FUNCTION "ASSE Y" : VOID
TITLE =GESTIONE SEGNALI DI STATO E COMANDO DELL'ASSE Y
VERSION : 0.1

BEGIN
NETWORK
TITLE =INS./DISIN.1
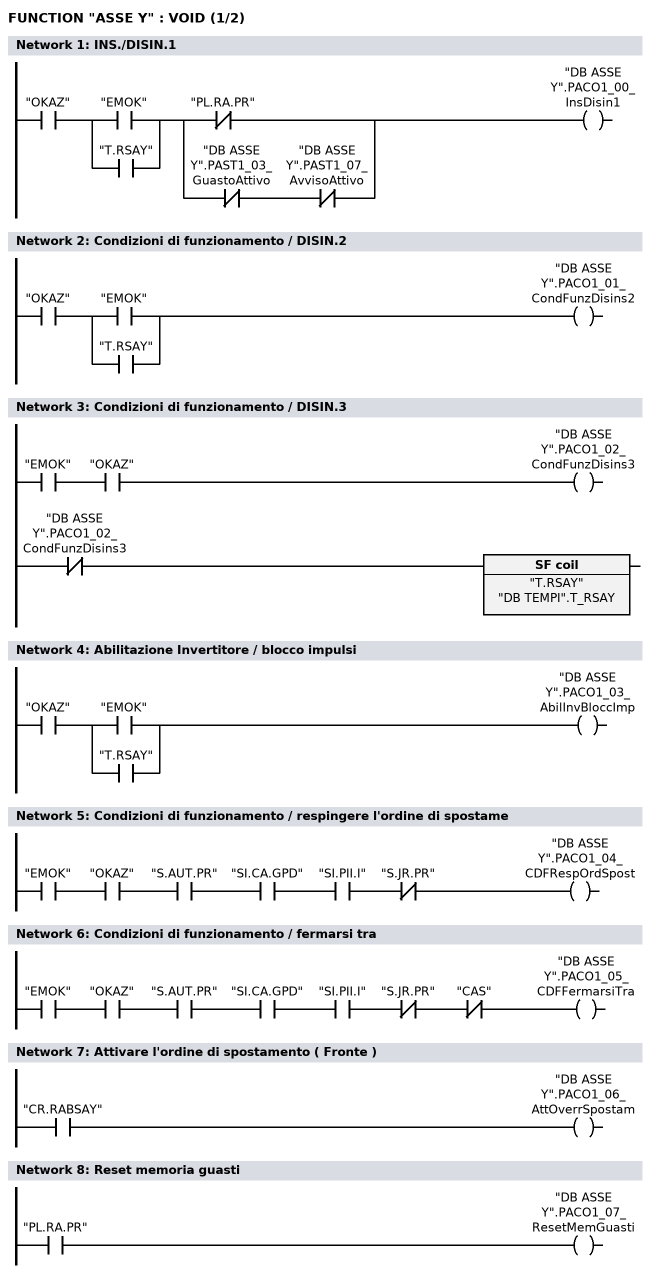
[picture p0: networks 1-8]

      U     "OKAZ";
      U(    ;
      O     "EMOK";
      O     "T.RSAY";
      )     ;
      U(    ;
      UN    "PL.RA.PR";
      O     ;
      UN    "DB ASSE Y".PAST1_03_GuastoAttivo;
      UN    "DB ASSE Y".PAST1_07_AvvisoAttivo;
      )     ;
      =     "DB ASSE Y".PACO1_00_InsDisin1;

NETWORK
TITLE =Condizioni di funzionamento / DISIN.2

      U     "OKAZ";
      U(    ;
      O     "EMOK";
      O     "T.RSAY";
      )     ;
      =     "DB ASSE Y".PACO1_01_CondFunzDisins2;

NETWORK
TITLE =Condizioni di funzionamento / DISIN.3

      U     "EMOK";
      U     "OKAZ";
      =     "DB ASSE Y".PACO1_02_CondFunzDisins3;
//---------------------------
      UN    "DB ASSE Y".PACO1_02_CondFunzDisins3;
      L     "DB TEMPI".T_RSAY;
      SA    "T.RSAY";

NETWORK
TITLE =Abilitazione Invertitore / blocco impulsi

      U     "OKAZ";
      U(    ;
      O     "EMOK";
      O     "T.RSAY";
      )     ;
      =     "DB ASSE Y".PACO1_03_AbilInvBloccImp;

NETWORK
TITLE =Condizioni di funzionamento / respingere l'ordine di spostame

      U     "EMOK";
      U     "OKAZ";
      U     "S.AUT.PR";
      U     "SI.CA.GPD";
      U     "SI.PII.I";
      UN    "S.JR.PR";
      =     "DB ASSE Y".PACO1_04_CDFRespOrdSpost;

NETWORK
TITLE =Condizioni di funzionamento / fermarsi tra

      U     "EMOK";
      U     "OKAZ";
      U     "S.AUT.PR";
      U     "SI.CA.GPD";
      U     "SI.PII.I";
      UN    "S.JR.PR";
      UN    "CAS";
      =     "DB ASSE Y".PACO1_05_CDFFermarsiTra;

NETWORK
TITLE =Attivare l'ordine di spostamento ( Fronte )

      U     "CR.RABSAY";
      =     "DB ASSE Y".PACO1_06_AttOverrSpostam;

NETWORK
TITLE =Reset memoria guasti

      U     "PL.RA.PR";
      =     "DB ASSE Y".PACO1_07_ResetMemGuasti;

NETWORK
TITLE =Marcia impulsi 1 INS
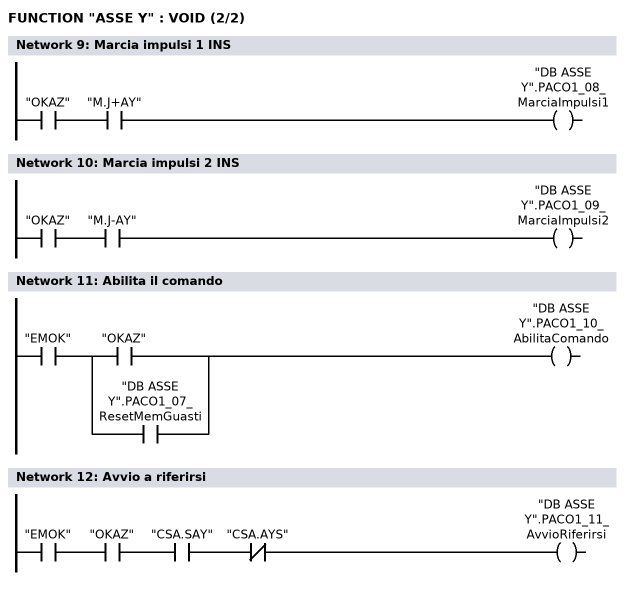
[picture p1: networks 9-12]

      U     "OKAZ";
      U     "M.J+AY";
      =     "DB ASSE Y".PACO1_08_MarciaImpulsi1;

NETWORK
TITLE =Marcia impulsi 2 INS

      U     "OKAZ";
      U     "M.J-AY";
      =     "DB ASSE Y".PACO1_09_MarciaImpulsi2;

NETWORK
TITLE =Abilita il comando

      U     "EMOK";
      U(    ;
      U     "OKAZ";
      O     ;
      U     "DB ASSE Y".PACO1_07_ResetMemGuasti;
      )     ;
      =     "DB ASSE Y".PACO1_10_AbilitaComando;

NETWORK
TITLE =Avvio a riferirsi

      U     "EMOK";
      U     "OKAZ";
      U     "CSA.SAY";
      UN    "CSA.AYS";
      =     "DB ASSE Y".PACO1_11_AvvioRiferirsi;

NETWORK
TITLE =Cambio del blocco esterno

      CLR   ;
      =     "DB ASSE Y".PACO1_13_CambioBloccoExt;

NETWORK
TITLE =Caricamento del numero blocco di spostamento desiderato



NETWORK
TITLE =Funzionamento a seguire
//
      CLR   ;
      =     "DB ASSE Y".POSPACO_00_FunzASeguire;

NETWORK
TITLE =Imposta il punto di riferimento

      CLR   ;
      =     "DB ASSE Y".POSPACO_01_ImpostPuntRif;

NETWORK
TITLE =Camma di riferimento

      UN    "E      47.5";
      =     "DB ASSE Y".POSPACO_02_CammaRiferime;

NETWORK
TITLE =Sensore della battuta fissa

      CLR   ;
      =     "DB ASSE Y".POSPACO_03_SensBattFissa;

NETWORK
TITLE =Attivare l'accoppiamento

      CLR   ;
      =     "DB ASSE Y".POSPACO_04_AttivAccoppia;

NETWORK
TITLE =Commutazione del blocco di parametri Bit 0

      CLR   ;
      =     "DB ASSE Y".PACO2_00_CommBlocParBit1;


NETWORK
TITLE =Commutazione del blocco di parametri Bit 1

      CLR   ;
      =     "DB ASSE Y".PACO2_01_CommBlocParBit2;

NETWORK
TITLE =Commutazione del blocco di parametri Bit 2

      CLR   ;
      =     "DB ASSE Y".PACO2_02_CommBlocParBit3;

NETWORK
TITLE =Primo filtro nel riferimento di velocita' disinserito
//
      CLR   ;
      =     "DB ASSE Y".PACO2_03_1FiltRifVelDisi;

NETWORK
TITLE =Tempo rampa zero

      CLR   ;
      =     "DB ASSE Y".PACO2_04_TempoRampaZero;

NETWORK
TITLE =Blocco dell'integratore nel regolatore di velocita'

      CLR   ;
      =     "DB ASSE Y".PACO2_06_BlocIntegrRegV;

NETWORK
TITLE =Scelta dell'asse in parcheggio

      CLR   ;
      =     "DB ASSE Y".PACO2_07_SceltaAsseInPar;

NETWORK
TITLE =Tacitare il guasto 608

      U     "OKAZ";
      U     "PL.RA.PR";
      =     "DB ASSE Y".PACO2_08_TacitGuasto608;

NETWORK
TITLE =Commutazione dati del motore 1 ingresso

      CLR   ;
      =     "DB ASSE Y".PACO2_09_CommDatiMot1Ing;

NETWORK
TITLE =Commutazione dati del motore 2 ingresso

      CLR   ;
      =     "DB ASSE Y".PACO2_10_CommDatiMot2Ing;

NETWORK
TITLE =Ha luogo la ommutazione del motore

      CLR   ;
      =     "DB ASSE Y".PACO2_11_CommutazMotore;

NETWORK
TITLE =OVERRIDE

      U     "M.MAN";
      UN    "P.JR.PR";
      SPBN  M001;
      L     "DB DATI".OVERRIDE_JOG;
      T     "DB ASSE Y".OVERRIDE;
      T     "DB DATI".OVERRIDE_ATTIVO;
M001: NOP   0;
      U     "M.MAN";
      U     "P.JR.PR";
      SPBN  M002;
      L     "DB DATI".OVERRIDE_JOG;
      L     2;
      *I    ;
      T     "DB ASSE Y".OVERRIDE;
      T     "DB DATI".OVERRIDE_ATTIVO;
M002: NOP   0;
      UN    "M.MAN";
      SPBN  M003;
      L     "DB DATI".OVERRIDE_AUT;
      T     "DB ASSE Y".OVERRIDE;
      T     "DB DATI".OVERRIDE_ATTIVO;
M003: NOP   0;

NETWORK
TITLE =Caricamento quote

      U     "ANSD";
      UN    "CQAY.IC";
      S     "CQAY.IC";
      S     "CQAY.Q1";
//============================ QUOTA 1
      U     "CQAY.Q1";
      SPBN  M004;
      L     W#16#8051;
      T     "DB ASSE Y".PKE_Scrittura;
      L     W#16#1;
      T     "DB ASSE Y".IND_Scrittura;
      L     "DB QUOTE".Y_ATTESA;
      T     DB122.DBD    4;
//----------------------------
      U(    ;
      L     "DB ASSE Y".PKE_Lettura;
      L     W#16#5051;
      ==I   ;
      )     ;
      U(    ;
      L     "DB ASSE Y".IND_Lettura;
      L     W#16#1;
      ==I   ;
      )     ;
      R     "CQAY.Q1";
      S     "CQAY.Q2";
M004: NOP   0;
//============================ QUOTA 2
      U     "CQAY.Q2";
      SPBN  M005;
      L     W#16#8051;
      T     "DB ASSE Y".PKE_Scrittura;
      L     W#16#2;
      T     "DB ASSE Y".IND_Scrittura;
      L     "DB QUOTE".Y_PRELIEVO;
      T     DB122.DBD    4;
//----------------------------
      U(    ;
      L     "DB ASSE Y".PKE_Lettura;
      L     W#16#5051;
      ==I   ;
      )     ;
      U(    ;
      L     "DB ASSE Y".IND_Lettura;
      L     W#16#2;
      ==I   ;
      )     ;
      R     "CQAY.Q2";
      S     "CQAY.Q3";
M005: NOP   0;
//============================ QUOTA 3
      U     "CQAY.Q3";
      SPBN  M006;
      L     W#16#8051;
      T     "DB ASSE Y".PKE_Scrittura;
      L     W#16#3;
      T     "DB ASSE Y".IND_Scrittura;
      L     "DB QUOTE".Y_DEPOSITO;
      T     DB122.DBD    4;
//----------------------------
      U(    ;
      L     "DB ASSE Y".PKE_Lettura;
      L     W#16#5051;
      ==I   ;
      )     ;
      U(    ;
      L     "DB ASSE Y".IND_Lettura;
      L     W#16#3;
      ==I   ;
      )     ;
      R     "CQAY.Q3";
      S     "CQAY.V1";
M006: NOP   0;
//============================ VELOCITA' 1
      U     "CQAY.V1";
      SPBN  M007;
      L     W#16#8052;
      T     "DB ASSE Y".PKE_Scrittura;
      L     W#16#1;
      T     "DB ASSE Y".IND_Scrittura;
      L     "DB QUOTE".VELOCITA_Y;
      T     DB122.DBD    4;
//----------------------------
      U(    ;
      L     "DB ASSE Y".PKE_Lettura;
      L     W#16#5052;
      ==I   ;
      )     ;
      U(    ;
      L     "DB ASSE Y".IND_Lettura;
      L     W#16#1;
      ==I   ;
      )     ;
      R     "CQAY.V1";
      S     "CQAY.V2";
M007: NOP   0;
//============================ VELOCITA' 2
      U     "CQAY.V2";
      SPBN  M008;
      L     W#16#8052;
      T     "DB ASSE Y".PKE_Scrittura;
      L     W#16#2;
      T     "DB ASSE Y".IND_Scrittura;
      L     "DB QUOTE".VELOCITA_Y;
      T     DB122.DBD    4;
//----------------------------
      U(    ;
      L     "DB ASSE Y".PKE_Lettura;
      L     W#16#5052;
      ==I   ;
      )     ;
      U(    ;
      L     "DB ASSE Y".IND_Lettura;
      L     W#16#2;
      ==I   ;
      )     ;
      R     "CQAY.V2";
      S     "CQAY.V3";
M008: NOP   0;
//============================ VELOCITA' 3
      U     "CQAY.V3";
      SPBN  M009;
      L     W#16#8052;
      T     "DB ASSE Y".PKE_Scrittura;
      L     W#16#3;
      T     "DB ASSE Y".IND_Scrittura;
      L     "DB QUOTE".VELOCITA_Y;
      T     DB122.DBD    4;
//----------------------------
      U(    ;
      L     "DB ASSE Y".PKE_Lettura;
      L     W#16#5052;
      ==I   ;
      )     ;
      U(    ;
      L     "DB ASSE Y".IND_Lettura;
      L     W#16#3;
      ==I   ;
      )     ;
      R     "CQAY.V3";
      S     "CQAY.CT";
M009: NOP   0;
      U     "CQAY.CT";
      UN    "ANSD";
      R     "CQAY.CT";
      R     "CQAY.IC";


NETWORK
TITLE =Riduzione percentuale del limite di coppia

      L     0;
      T     "DB ASSE Y".MOMRID;

END_FUNCTION

